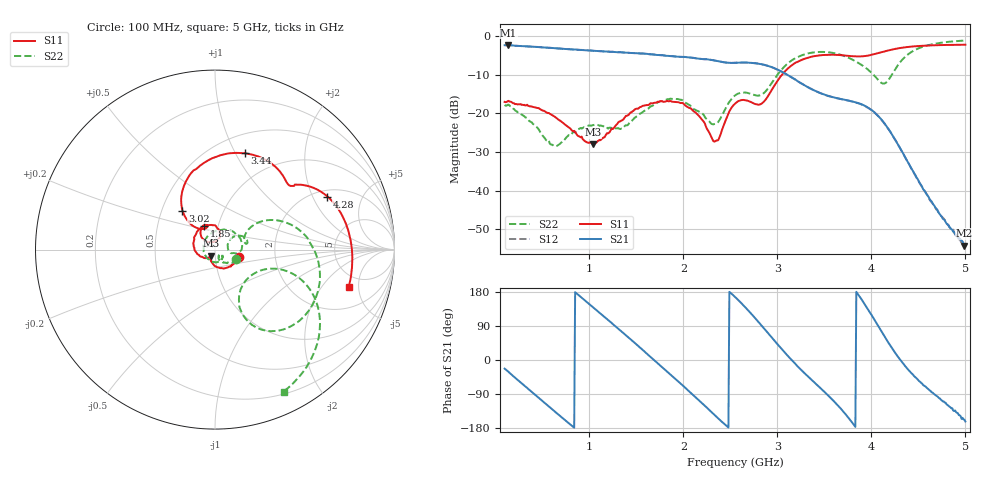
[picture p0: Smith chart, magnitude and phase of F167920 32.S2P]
!  2-Port S-parameters saved by WinCal
! VAR MeasName=S-Parameters (CALIBRATED_DATA) read from VNA (N5242A)
! VAR MeasDate=2016-11-22 9:56:44
! VAR NAME=F167920 32
! VAR FILENAME=F167920 32.S2P
! VAR DATE=2016-11-22 9:56:44
! VAR PHYS_PORTS=1,2
# Hz S DB R 50
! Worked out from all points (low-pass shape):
!   491 points, 100 MHz to 5 GHz, reference 50 ohm
!   highest |S21| = -2.32 dB at 140 MHz (marker M1); lowest = -54.2 dB at 4.99 GHz (marker M2)
!   |S21| within 3 dB of the highest: start of sweep to 1.932 GHz
!   lowest |S11| = -28.0 dB at 1.04 GHz (marker M3), VSWR 1.08, Z = 47.8 - j3.23 ohm
!   |S11| at or under -10 dB: start of sweep to 3.05 GHz
!   |S22| runs from -28.5 to -1.1 dB; largest |S21 - S12| = 0.00097
!   S11 on the Smith chart (normalised r, x): 100 MHz: 1.30, -0.11; 1.85 GHz: 0.86, +0.23; 3.02 GHz: 0.64, +0.30; 3.44 GHz: 0.69, +1.09; 4.28 GHz: 2.29, +2.61; 5 GHz: 3.70, -3.84
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1e8  -17.03 -17.8  -2.35 -22.8  -2.35 -22.8  -17.83 -23.6
1.4e8  -16.76 -20.9  -2.32 -31.1  -2.31 -31.1  -17.72 -27.9
4.7e8  -18.80 -66.5  -2.83 -101.5  -2.83 -101.5  -24.42 -68.1
6.4e8  -21.01 -92.3  -3.14 -137.3  -3.14 -137.3  -28.55 -48.8
9.2e8  -26.01 -122.2  -3.58 164.5  -3.57 164.5  -23.95 -54.4
1.04e9  -28.00 -122.1  -3.78 139.1  -3.78 139.1  -23.04 -75.2
1.34e9  -21.89 -148.6  -4.19 75.8  -4.20 75.8  -23.97 176.4
1.74e9  -17.00 133.0  -4.90 -11.1  -4.90 -11.2  -17.06 46.6
1.85e9  -16.87 114.6  -5.15 -35.2  -5.16 -35.3  -16.30 25.3
2.09e9  -18.93 78.7  -5.58 -89.1  -5.58 -89.2  -18.43 -10.6
2.34e9  -27.22 102.3  -6.35 -147.1  -6.36 -147.1  -22.70 12.5
2.55e9  -17.53 126.8  -6.90 166.6  -6.90 166.5  -15.37 26.1
2.8e9  -17.76 114.6  -7.14 100.4  -7.14 100.3  -15.41 16.3
3.02e9  -10.96 129.9  -8.87 36.6  -8.88 36.4  -9.41 29.0
3.37e9  -5.30 81.3  -13.78 -53.6  -13.80 -53.7  -4.27 -17.6
3.44e9  -5.01 73.0  -14.56 -69.8  -14.60 -69.8  -4.11 -26.3
3.75e9  -5.10 46.1  -16.66 -150.4  -16.67 -150.3  -5.52 -58.3
4.19e9  -3.65 30.9  -24.33 42.4  -24.35 42.5  -11.08 -24.7
4.28e9  -3.19 25.3  -27.91 9.4  -27.91 9.7  -7.61 -16.7
4.53e9  -2.52 9.2  -38.59 -60.6  -38.74 -60.3  -2.89 -35.3
4.99e9  -2.23 -15.2  -54.23 -157.7  -54.09 -160.1  -1.14 -63.8
5e9  -2.23 -15.7  -53.97 -162.2  -54.39 -162.8  -1.13 -64.2
